FUNCTION "STATUS_OP_DB" : VOID
TITLE =BLOCK DATA BEETWEN OP_37 AND PLC
AUTHOR : Esposito
FAMILY : EGAL_srl
NAME : MONITOR
VERSION : 0.1

BEGIN
NETWORK
TITLE =MONITOR ALARM
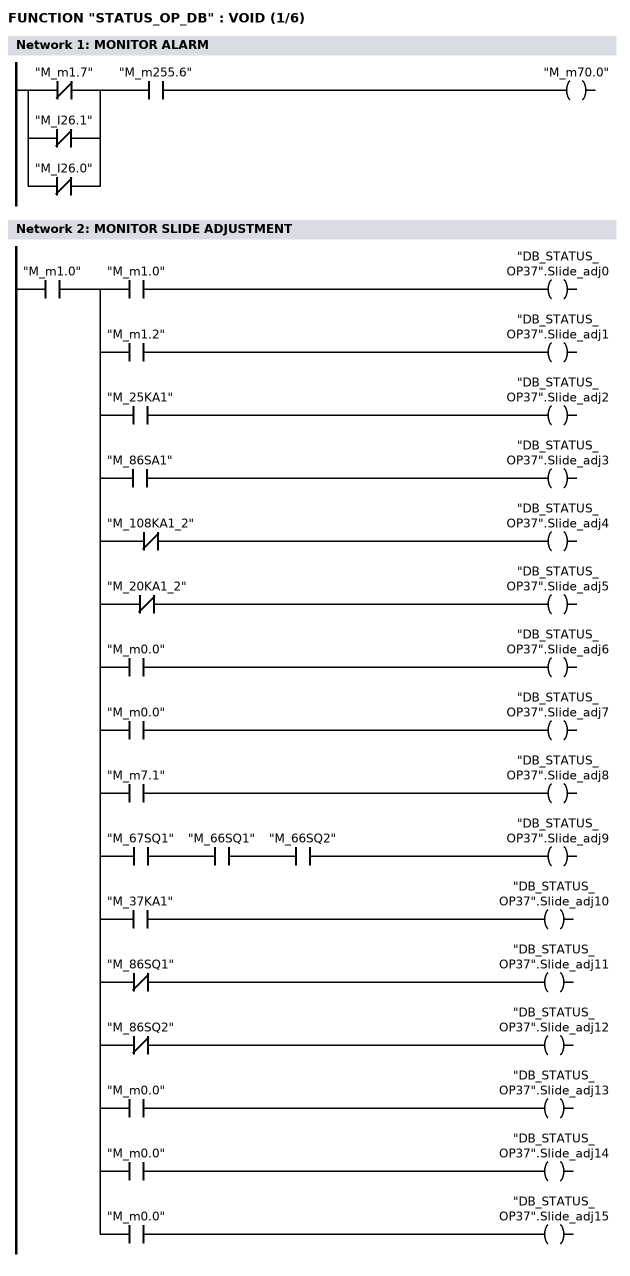
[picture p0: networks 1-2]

      U(    ;
      ON    "M_m1.7";
      ON    "M_I26.1";
      ON    "M_I26.0";
      )     ;
      U     "M_m255.6";
      =     "M_m70.0";
NETWORK
TITLE =MONITOR SLIDE ADJUSTMENT

      U     "M_m1.0";
      =     L      0.0;
      U     L      0.0;
      U     "M_m1.0";
      =     "DB_STATUS_OP37".Slide_adj0;
      U     L      0.0;
      U     "M_m1.2";
      =     "DB_STATUS_OP37".Slide_adj1;
      U     L      0.0;
      U     "M_25KA1";
      =     "DB_STATUS_OP37".Slide_adj2;
      U     L      0.0;
      U     "M_86SA1";
      =     "DB_STATUS_OP37".Slide_adj3;
      U     L      0.0;
      UN    "M_108KA1_2";
      =     "DB_STATUS_OP37".Slide_adj4;
      U     L      0.0;
      UN    "M_20KA1_2";
      =     "DB_STATUS_OP37".Slide_adj5;
      U     L      0.0;
      U     "M_m0.0";
      =     "DB_STATUS_OP37".Slide_adj6;
      U     L      0.0;
      U     "M_m0.0";
      =     "DB_STATUS_OP37".Slide_adj7;
      U     L      0.0;
      U     "M_m7.1";
      =     "DB_STATUS_OP37".Slide_adj8;
      U     L      0.0;
      U     "M_67SQ1";
      U     "M_66SQ1";
      U     "M_66SQ2";
      =     "DB_STATUS_OP37".Slide_adj9;
      U     L      0.0;
      U     "M_37KA1";
      =     "DB_STATUS_OP37".Slide_adj10;
      U     L      0.0;
      UN    "M_86SQ1";
      =     "DB_STATUS_OP37".Slide_adj11;
      U     L      0.0;
      UN    "M_86SQ2";
      =     "DB_STATUS_OP37".Slide_adj12;
      U     L      0.0;
      U     "M_m0.0";
      =     "DB_STATUS_OP37".Slide_adj13;
      U     L      0.0;
      U     "M_m0.0";
      =     "DB_STATUS_OP37".Slide_adj14;
      U     L      0.0;
      U     "M_m0.0";
      =     "DB_STATUS_OP37".Slide_adj15;
NETWORK
TITLE =MONITOR LUBRICATION
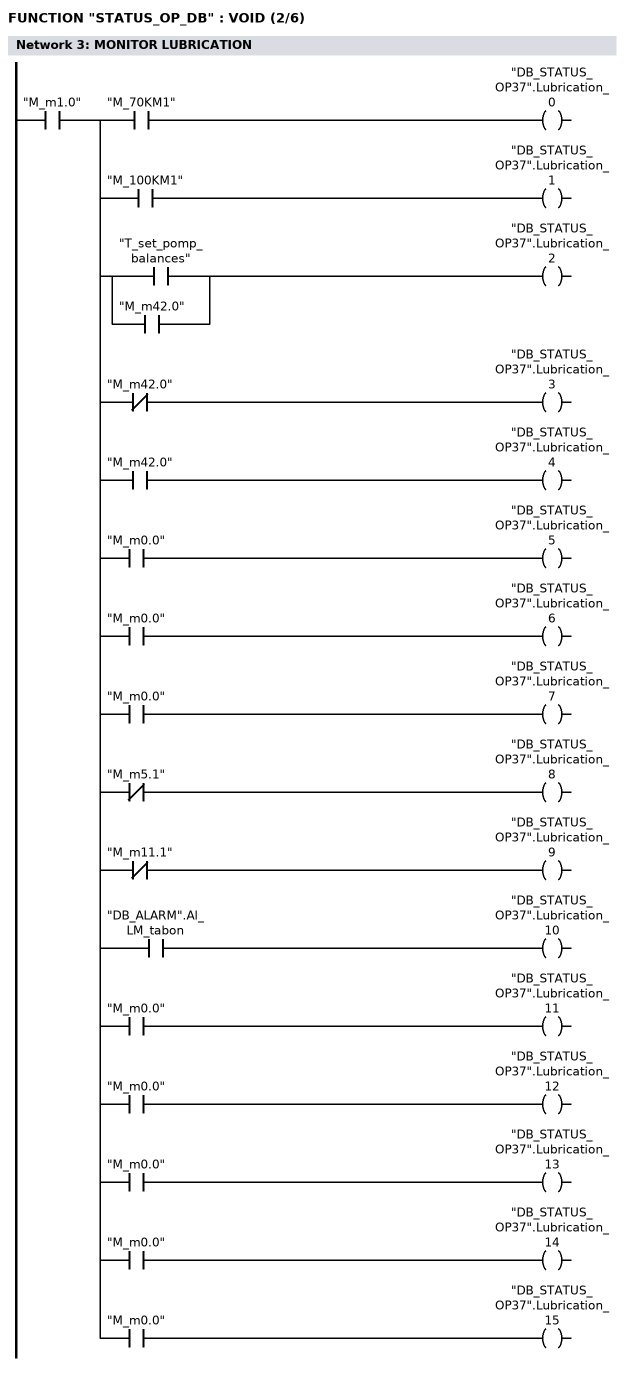
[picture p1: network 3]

      U     "M_m1.0";
      =     L      0.0;
      U     L      0.0;
      U     "M_70KM1";
      =     "DB_STATUS_OP37".Lubrication_0;
      U     L      0.0;
      U     "M_100KM1";
      =     "DB_STATUS_OP37".Lubrication_1;
      U     L      0.0;
      U(    ;
      O     "T_set_pomp_balances";
      O     "M_m42.0";
      )     ;
      =     "DB_STATUS_OP37".Lubrication_2;
      U     L      0.0;
      UN    "M_m42.0";
      =     "DB_STATUS_OP37".Lubrication_3;
      U     L      0.0;
      U     "M_m42.0";
      =     "DB_STATUS_OP37".Lubrication_4;
      U     L      0.0;
      U     "M_m0.0";
      =     "DB_STATUS_OP37".Lubrication_5;
      U     L      0.0;
      U     "M_m0.0";
      =     "DB_STATUS_OP37".Lubrication_6;
      U     L      0.0;
      U     "M_m0.0";
      =     "DB_STATUS_OP37".Lubrication_7;
      U     L      0.0;
      UN    "M_m5.1";
      =     "DB_STATUS_OP37".Lubrication_8;
      U     L      0.0;
      UN    "M_m11.1";
      =     "DB_STATUS_OP37".Lubrication_9;
      U     L      0.0;
      U     "DB_ALARM".Al_LM_tabon;
      =     "DB_STATUS_OP37".Lubrication_10;
      U     L      0.0;
      U     "M_m0.0";
      =     "DB_STATUS_OP37".Lubrication_11;
      U     L      0.0;
      U     "M_m0.0";
      =     "DB_STATUS_OP37".Lubrication_12;
      U     L      0.0;
      U     "M_m0.0";
      =     "DB_STATUS_OP37".Lubrication_13;
      U     L      0.0;
      U     "M_m0.0";
      =     "DB_STATUS_OP37".Lubrication_14;
      U     L      0.0;
      U     "M_m0.0";
      =     "DB_STATUS_OP37".Lubrication_15;
NETWORK
TITLE =MONITOR OVERLOAD
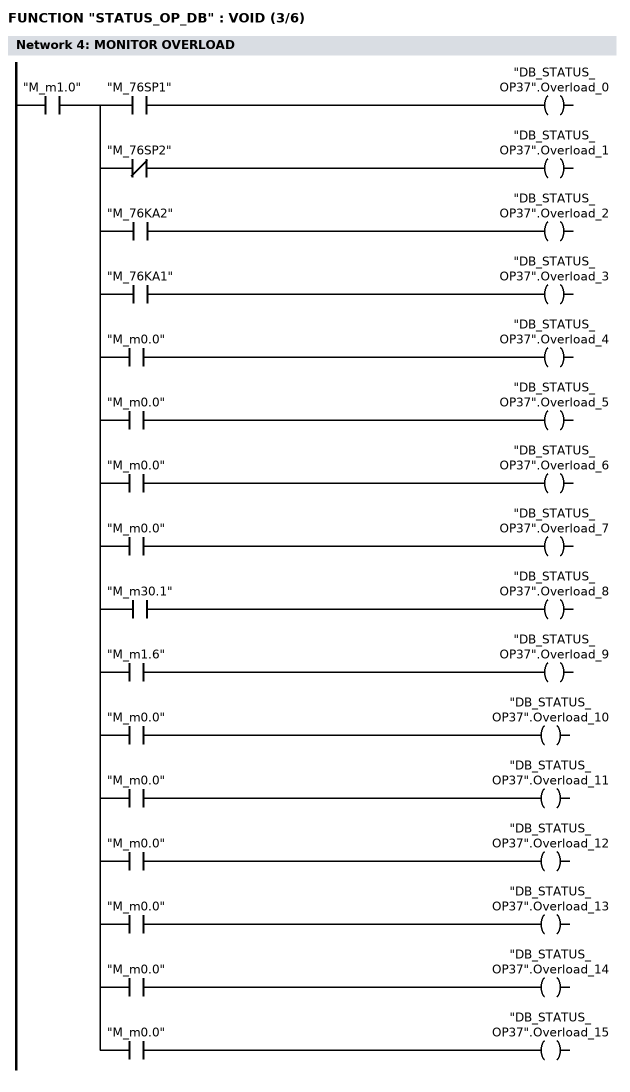
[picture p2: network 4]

      U     "M_m1.0";
      =     L      0.0;
      U     L      0.0;
      U     "M_76SP1";
      =     "DB_STATUS_OP37".Overload_0;
      U     L      0.0;
      UN    "M_76SP2";
      =     "DB_STATUS_OP37".Overload_1;
      U     L      0.0;
      U     "M_76KA2";
      =     "DB_STATUS_OP37".Overload_2;
      U     L      0.0;
      U     "M_76KA1";
      =     "DB_STATUS_OP37".Overload_3;
      U     L      0.0;
      U     "M_m0.0";
      =     "DB_STATUS_OP37".Overload_4;
      U     L      0.0;
      U     "M_m0.0";
      =     "DB_STATUS_OP37".Overload_5;
      U     L      0.0;
      U     "M_m0.0";
      =     "DB_STATUS_OP37".Overload_6;
      U     L      0.0;
      U     "M_m0.0";
      =     "DB_STATUS_OP37".Overload_7;
      U     L      0.0;
      U     "M_m30.1";
      =     "DB_STATUS_OP37".Overload_8;
      U     L      0.0;
      U     "M_m1.6";
      =     "DB_STATUS_OP37".Overload_9;
      U     L      0.0;
      U     "M_m0.0";
      =     "DB_STATUS_OP37".Overload_10;
      U     L      0.0;
      U     "M_m0.0";
      =     "DB_STATUS_OP37".Overload_11;
      U     L      0.0;
      U     "M_m0.0";
      =     "DB_STATUS_OP37".Overload_12;
      U     L      0.0;
      U     "M_m0.0";
      =     "DB_STATUS_OP37".Overload_13;
      U     L      0.0;
      U     "M_m0.0";
      =     "DB_STATUS_OP37".Overload_14;
      U     L      0.0;
      U     "M_m0.0";
      =     "DB_STATUS_OP37".Overload_15;
NETWORK
TITLE =MONITOR BALANCING
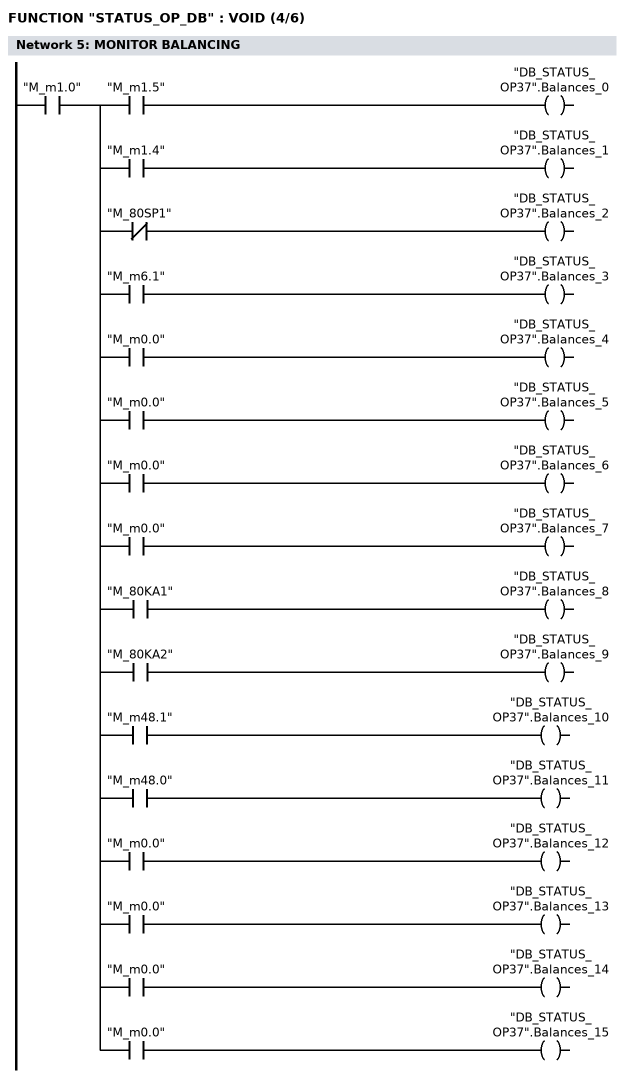
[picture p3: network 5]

      U     "M_m1.0";
      =     L      0.0;
      U     L      0.0;
      U     "M_m1.5";
      =     "DB_STATUS_OP37".Balances_0;
      U     L      0.0;
      U     "M_m1.4";
      =     "DB_STATUS_OP37".Balances_1;
      U     L      0.0;
      UN    "M_80SP1";
      =     "DB_STATUS_OP37".Balances_2;
      U     L      0.0;
      U     "M_m6.1";
      =     "DB_STATUS_OP37".Balances_3;
      U     L      0.0;
      U     "M_m0.0";
      =     "DB_STATUS_OP37".Balances_4;
      U     L      0.0;
      U     "M_m0.0";
      =     "DB_STATUS_OP37".Balances_5;
      U     L      0.0;
      U     "M_m0.0";
      =     "DB_STATUS_OP37".Balances_6;
      U     L      0.0;
      U     "M_m0.0";
      =     "DB_STATUS_OP37".Balances_7;
      U     L      0.0;
      U     "M_80KA1";
      =     "DB_STATUS_OP37".Balances_8;
      U     L      0.0;
      U     "M_80KA2";
      =     "DB_STATUS_OP37".Balances_9;
      U     L      0.0;
      U     "M_m48.1";
      =     "DB_STATUS_OP37".Balances_10;
      U     L      0.0;
      U     "M_m48.0";
      =     "DB_STATUS_OP37".Balances_11;
      U     L      0.0;
      U     "M_m0.0";
      =     "DB_STATUS_OP37".Balances_12;
      U     L      0.0;
      U     "M_m0.0";
      =     "DB_STATUS_OP37".Balances_13;
      U     L      0.0;
      U     "M_m0.0";
      =     "DB_STATUS_OP37".Balances_14;
      U     L      0.0;
      U     "M_m0.0";
      =     "DB_STATUS_OP37".Balances_15;
NETWORK
TITLE =MONITOR INLETS
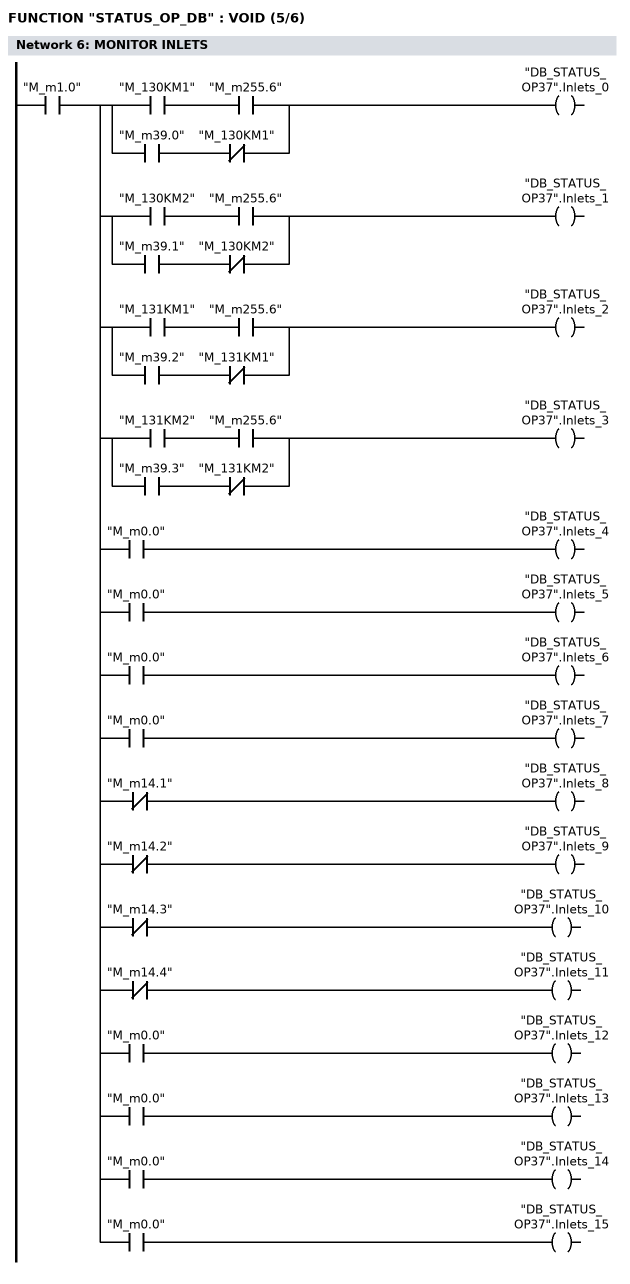
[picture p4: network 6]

      U     "M_m1.0";
      =     L      0.0;
      U     L      0.0;
      U(    ;
      U     "M_130KM1";
      U     "M_m255.6";
      O     ;
      U     "M_m39.0";
      UN    "M_130KM1";
      )     ;
      =     "DB_STATUS_OP37".Inlets_0;
      U     L      0.0;
      U(    ;
      U     "M_130KM2";
      U     "M_m255.6";
      O     ;
      U     "M_m39.1";
      UN    "M_130KM2";
      )     ;
      =     "DB_STATUS_OP37".Inlets_1;
      U     L      0.0;
      U(    ;
      U     "M_131KM1";
      U     "M_m255.6";
      O     ;
      U     "M_m39.2";
      UN    "M_131KM1";
      )     ;
      =     "DB_STATUS_OP37".Inlets_2;
      U     L      0.0;
      U(    ;
      U     "M_131KM2";
      U     "M_m255.6";
      O     ;
      U     "M_m39.3";
      UN    "M_131KM2";
      )     ;
      =     "DB_STATUS_OP37".Inlets_3;
      U     L      0.0;
      U     "M_m0.0";
      =     "DB_STATUS_OP37".Inlets_4;
      U     L      0.0;
      U     "M_m0.0";
      =     "DB_STATUS_OP37".Inlets_5;
      U     L      0.0;
      U     "M_m0.0";
      =     "DB_STATUS_OP37".Inlets_6;
      U     L      0.0;
      U     "M_m0.0";
      =     "DB_STATUS_OP37".Inlets_7;
      U     L      0.0;
      UN    "M_m14.1";
      =     "DB_STATUS_OP37".Inlets_8;
      U     L      0.0;
      UN    "M_m14.2";
      =     "DB_STATUS_OP37".Inlets_9;
      U     L      0.0;
      UN    "M_m14.3";
      =     "DB_STATUS_OP37".Inlets_10;
      U     L      0.0;
      UN    "M_m14.4";
      =     "DB_STATUS_OP37".Inlets_11;
      U     L      0.0;
      U     "M_m0.0";
      =     "DB_STATUS_OP37".Inlets_12;
      U     L      0.0;
      U     "M_m0.0";
      =     "DB_STATUS_OP37".Inlets_13;
      U     L      0.0;
      U     "M_m0.0";
      =     "DB_STATUS_OP37".Inlets_14;
      U     L      0.0;
      U     "M_m0.0";
      =     "DB_STATUS_OP37".Inlets_15;
NETWORK
TITLE =MONITOR ROBOT
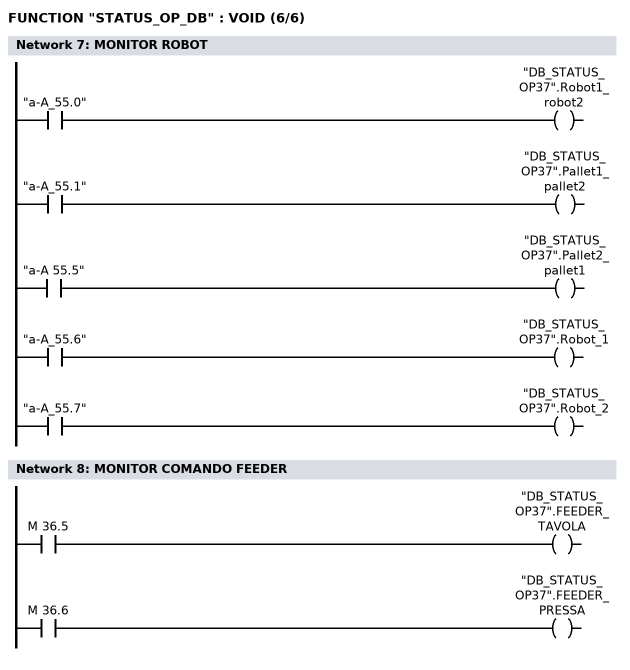
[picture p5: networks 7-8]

      U     "a-A_55.0";
      =     "DB_STATUS_OP37".Robot1_robot2;

      U     "a-A_55.1";
      =     "DB_STATUS_OP37".Pallet1_pallet2;

      U     "a-A 55.5";
      =     "DB_STATUS_OP37".Pallet2_pallet1;

      U     "a-A_55.6";
      =     "DB_STATUS_OP37".Robot_1;

      U     "a-A_55.7";
      =     "DB_STATUS_OP37".Robot_2;

NETWORK
TITLE =MONITOR COMANDO FEEDER

      U     M     36.5;
      =     "DB_STATUS_OP37".FEEDER_TAVOLA;

      U     M     36.6;
      =     "DB_STATUS_OP37".FEEDER_PRESSA;


END_FUNCTION

